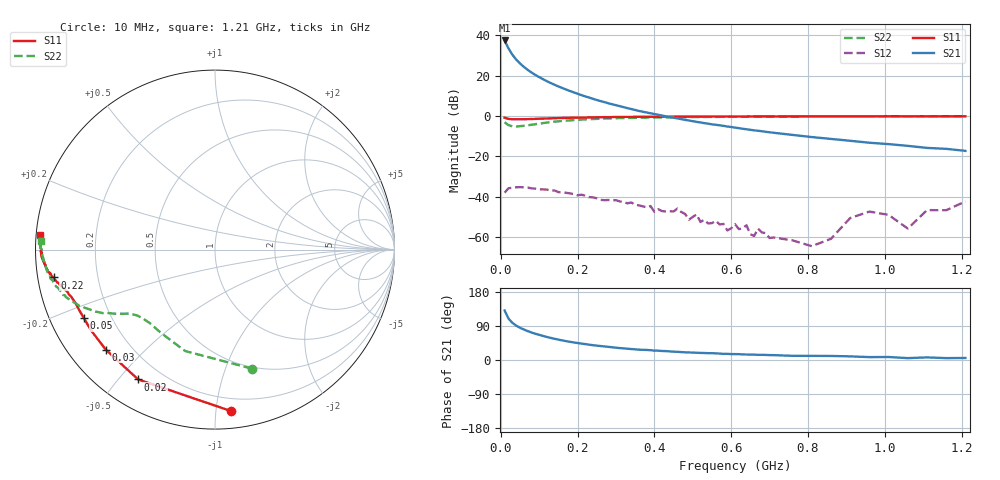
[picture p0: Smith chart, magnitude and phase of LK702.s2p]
! Date: Wed May 20 11:25:11 1998
!  POLYFET RF DEVICES
!  LP702/LK702
!  28Vdc		400ma
# MHZ  S  MA  R  50.0000
! SCATTERING PARAMETERS :
! Freq=MHz Mag[s11] Ang[s11] Mag[s21] Ang[s21] Mag[s12] Ang[s12] Mag[s22] Ang[s22]
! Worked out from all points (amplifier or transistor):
!   81 points, 10 MHz to 1.21 GHz, reference 50 ohm
!   highest |S21| = 37.4 dB at 10 MHz (marker M1)
!   |S21| within 3 dB of that: start of sweep to 17.69 MHz
!   unconditionally stable (mu >= 1): 397.9 MHz to 403.4 MHz; 439.7 MHz to 450.6 MHz; 475.1 MHz to end of sweep
!   at 140 MHz: K = 0.11, MSG = 26.2 dB, |S12| = -37.0 dB
!   at 410 MHz: K = 0.69, MSG = 23.4 dB, |S12| = -46.3 dB
!   at 1.21 GHz: K = 1.80, MAG = 7.3 dB, |S12| = -42.4 dB
!   S11 on the Smith chart (normalised r, x): 10 MHz: 0.11, -1.10; 20 MHz: 0.11, -0.56; 30 MHz: 0.11, -0.38; 50 MHz: 0.10, -0.24; 220 MHz: 0.05, -0.09; 1.21 GHz: 0.01, +0.04
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10  0.9033 -84.4  74.05 130.7  0.01248 38.7  0.6946 -72.7
20  0.8407 -120.7  47.26 109.5  0.01607 19.2  0.589 -106.4
30  0.8252 -137.5  33.07 98.3  0.0165 9.6  0.5534 -122.8
40  0.8244 -146.9  25 90.9  0.017 1.9  0.5475 -131.6
50  0.8244 -152.4  19.98 85.1  0.01712 -3.3  0.5559 -136.4
60  0.8282 -155.9  16.44 80.5  0.01696 -6.7  0.5674 -139.7
70  0.8312 -158.5  13.85 76.3  0.01678 -10.5  0.5845 -141.9
80  0.8368 -160.3  11.9 72.5  0.016 -16.3  0.6021 -143.7
100  0.8515 -162.9  9.143 66.4  0.01512 -19.0  0.6423 -146.2
120  0.8634 -164.8  7.259 60.8  0.01491 -24.0  0.6807 -148.6
150  0.8813 -166.7  5.384 53.8  0.01286 -32.7  0.7334 -151.6
210  0.9103 -169.7  3.276 43.3  0.01113 -39.3  0.8084 -157.1
220  0.9081 -170.2  3.041 41.9  0.01056 -39.1  0.8198 -157.5
300  0.9386 -172.5  1.84 32.5  0.00814 -48.7  0.8736 -163.0
410  0.9544 -175.2  1.064 24.6  0.00486 -42.0  0.9145 -168.4
610  0.966 -178.3  0.5129 15.6  0.00208 -62.1  0.9471 -174.0
810  0.9736 179.3  0.2986 10.8  0.00059 173.3  0.9624 -178.0
910  0.9732 178.2  0.2416 9.6  0.00294 127.6  0.9655 -179.2
1010  0.9763 177.4  0.1996 7.9  0.00352 121.6  0.974 179.4
1060  0.9753 176.7  0.1806 4.9  0.00161 119.8  0.9726 178.8
1110  0.9765 176.3  0.1609 6.9  0.00462 138.8  0.9704 178.0
1210  0.9763 175.3  0.1358 5.4  0.00759 113.0  0.9723 177.1
